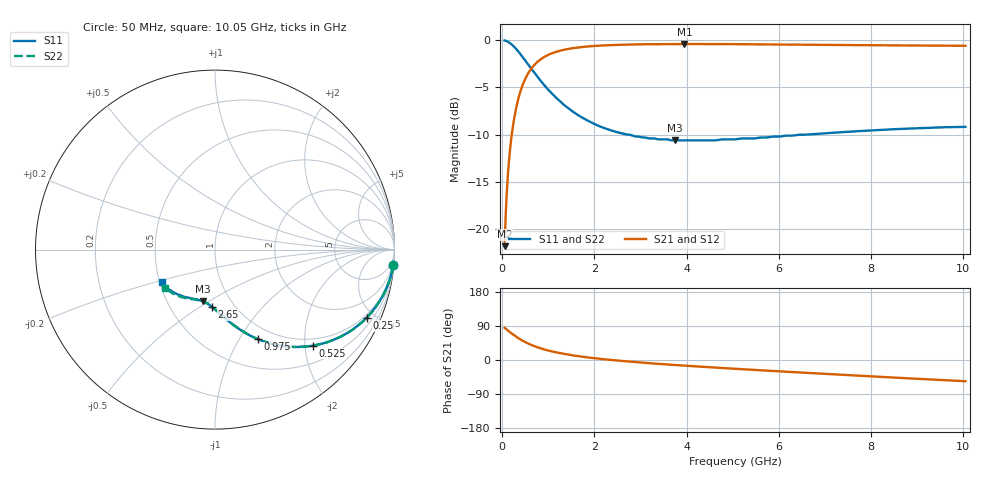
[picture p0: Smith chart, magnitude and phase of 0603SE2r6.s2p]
! AVX Thin Film Operation		Date: August 2001
! Description: Accu-P® Series, Thin Film, SMD, RF Capacitor
! Part Number: 06035J2R6ABT
! 50 MHz  -  10.05 GHz
! Serial Measurements
# mhz S db R 50
!	S11		S21		S12		S22
!	dB	Phase	dB	Phase	dB	Phase	dB	Phase
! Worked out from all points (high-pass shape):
!   401 points, 50 MHz to 10.05 GHz, reference 50 ohm
!   highest |S21| = -0.41 dB at 3.95 GHz (marker M1); lowest = -21.8 dB at 50 MHz (marker M2)
!   |S21| within 3 dB of the highest: 573.9 MHz to end of sweep
!   lowest |S11| = -10.6 dB at 3.75 GHz (marker M3), VSWR 1.84, Z = 37.3 - j23.5 ohm
!   |S11| at or under -10 dB: 2.754 GHz to 6.45 GHz (3.696 GHz wide, 80.3 % of centre); 6.475 GHz to 6.575 GHz (100 MHz wide, 1.53 % of centre)
!   |S22| runs from -10.6 to 0.0 dB; largest |S21 - S12| = 0
!   S11 on the Smith chart (normalised r, x): 50 MHz: 1, -23; 250 MHz: 0.84, -4.52; 525 MHz: 0.85, -2.18; 975 MHz: 0.84, -1.21; 2.65 GHz: 0.79, -0.56; 10.05 GHz: 0.51, -0.21
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50  -0.03 -5.1  -21.80 84.9  -21.80 84.9  -0.03 -5.1
75  -0.07 -7.6  -18.31 82.4  -18.31 82.4  -0.07 -7.6
125  -0.18 -12.6  -13.98 77.4  -13.98 77.4  -0.18 -12.6
150  -0.25 -15.0  -12.50 75.0  -12.50 75.0  -0.25 -15.0
200  -0.44 -19.6  -10.17 70.3  -10.17 70.3  -0.44 -19.6
250  -0.67 -24.2  -8.49 65.8  -8.49 65.8  -0.67 -24.2
300  -0.93 -28.4  -7.18 61.6  -7.18 61.6  -0.93 -28.4
375  -1.36 -34.3  -5.71 55.7  -5.71 55.7  -1.36 -34.3
525  -2.33 -44.4  -3.83 45.6  -3.83 45.6  -2.33 -44.4
725  -3.64 -54.8  -2.47 35.2  -2.47 35.2  -3.64 -54.7
975  -5.12 -64.2  -1.61 25.7  -1.61 25.7  -5.11 -64.2
1350  -6.89 -74.2  -1.00 15.8  -1.00 15.8  -6.89 -74.0
1725  -8.16 -81.1  -0.73 8.9  -0.73 8.9  -8.16 -80.9
2150  -9.19 -87.4  -0.57 2.7  -0.57 2.7  -9.18 -87.0
2650  -9.92 -93.1  -0.47 -3.0  -0.47 -3.0  -9.92 -92.6
3400  -10.50 -100.3  -0.42 -10.3  -0.42 -10.3  -10.50 -99.6
3750  -10.60 -103.3  -0.41 -13.2  -0.41 -13.2  -10.60 -102.3
3950  -10.60 -105.1  -0.41 -14.9  -0.41 -14.9  -10.60 -104.1
5050  -10.50 -114.0  -0.42 -23.2  -0.42 -23.2  -10.50 -112.0
6725  -9.95 -126.0  -0.48 -34.7  -0.48 -34.7  -9.93 -123.0
8400  -9.45 -138.1  -0.55 -45.7  -0.55 -45.7  -9.41 -133.1
10050  -9.17 -148.6  -0.59 -56.0  -0.59 -56.0  -9.13 -142.8
